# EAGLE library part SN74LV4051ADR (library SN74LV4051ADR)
8-Channel Analog Multiplexer/Demultiplexer Source: Datasheet
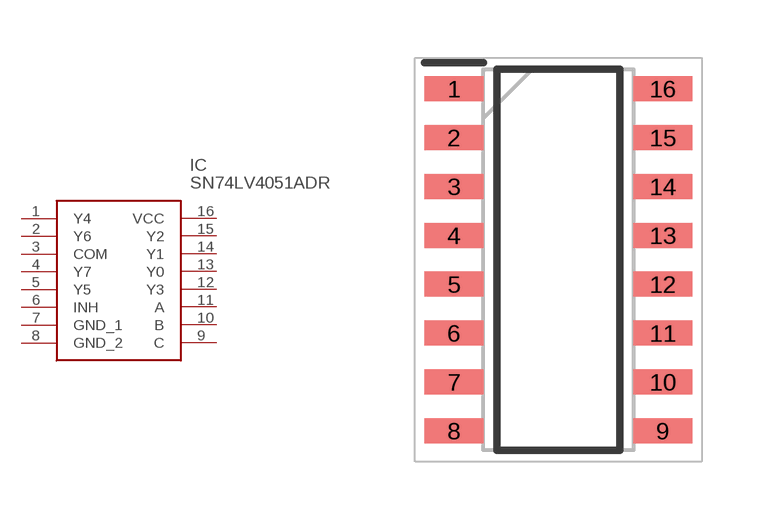
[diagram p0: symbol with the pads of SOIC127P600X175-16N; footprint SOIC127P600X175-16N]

Designator prefix IC

## SN74LV4051ADR (Description: 8-Channel Analog Multiplexer/Demultiplexer; Height: 1.75mm; Manufacturer_Name: Texas Instruments; Manufacturer_Part_Number: SN74LV4051ADR; Mouser_Part_Number: 595-SN74LV4051ADR; Mouser_Price-Stock: https://www.mouser.co.uk/ProductDetail/Texas-Instruments/SN74LV4051ADR?qs=8Pd2FuFSoMHt2f%2FU0%252B0rVg%3D%3D)  [SOIC127P600X175-16N]
1  Y4
2  Y6
3  COM
4  Y7
5  Y5
6  INH
7  GND_1
8  GND_2
9  C
10  B
11  A
12  Y3
13  Y0
14  Y1
15  Y2
16  VCC

## Footprint SOIC127P600X175-16N (pad centres in mm)
D (R-PDSO-G16)
smd 1.525 x 0.65: 1 -2.712,4.445; 2 -2.712,3.175; 3 -2.712,1.905; 4 -2.712,0.635; 5 -2.712,-0.635; 6 -2.712,-1.905; 7 -2.712,-3.175; 8 -2.712,-4.445; 9 2.712,-4.445; 10 2.712,-3.175; 11 2.712,-1.905; 12 2.712,-0.635; 13 2.712,0.635; 14 2.712,1.905; 15 2.712,3.175; 16 2.712,4.445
